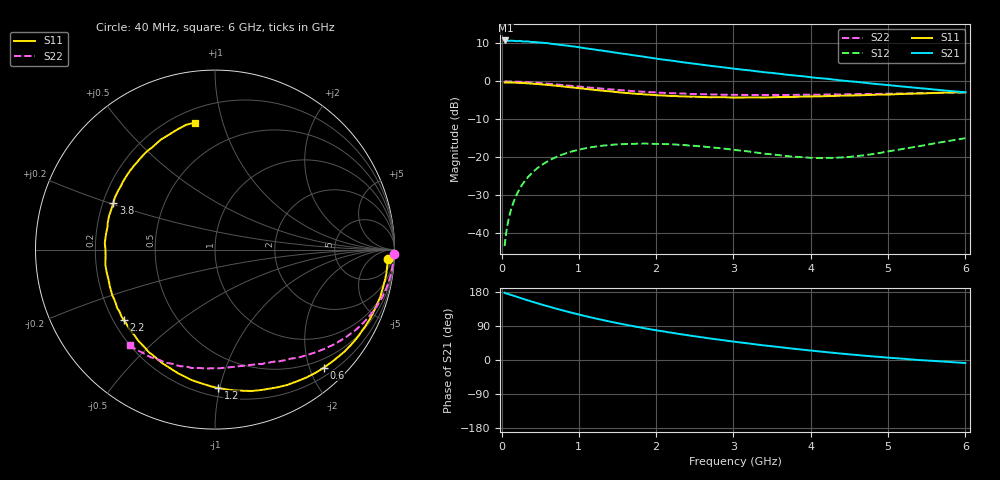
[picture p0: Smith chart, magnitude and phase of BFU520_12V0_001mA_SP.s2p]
! Filename:  P:\Prog\Test\Noise\ATS_data\Testdata_Net\03 Spar\BFU520_APG2013_37_A05_12p0V_001mA_SP_CM01_D.s2p
! Date/Time: Fri 26/Apr/2013 13:00:10
! BFU520_APG2013_37_A05_12p0V_1to20mA_SP_CM01_Bias1_R.s2p
! MDIF S-parameter v. bias file
! BFU520_APG2013_37_A05_12p0V_1to20mA_SP_CM01
! Date/time Tue Apr 23 18:22:57 2013
! bias mode 1
! bias variable = I_out
! VAR bias_var= 1
! VAR V_out= 12.0000
! VAR I_out= 0.9950
! VAR V_in= 0.7863
! VAR I_in= 0.0086
! Device data file deembeded for feedlines and parallel
! Original file: \03 Spar\BFU520_APG2013_37_A05_12p0V_001mA_SP_CM01_R.s2p
! Feed-files: PR047V01_250413_Feed1.s2p, PR047V01_250413_Feed2.s2p
! Parallel-file: PR047V01_250413_Par.s2p
# MHz S MA R 50
!  Freq-MHz  S11-mag  S11-arg  S21-mag  S21-arg  S12-mag  S12-arg  S22-mag  S22-arg
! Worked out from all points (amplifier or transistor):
!   98 points, 40 MHz to 6 GHz, reference 50 ohm
!   highest |S21| = 10.8 dB at 50 MHz (marker M1)
!   |S21| within 3 dB of that: start of sweep to 1.409 GHz
!   unconditionally stable (mu >= 1): 3.535 GHz to 5.175 GHz
!   at 300 MHz: K = 0.08, MSG = 18.4 dB, |S12| = -26.3 dB
!   at 1.6 GHz: K = 0.38, MSG = 11.9 dB, |S12| = -16.5 dB
!   at 6 GHz: K = 0.79, MSG = 6.1 dB, |S12| = -15.0 dB
!   S11 on the Smith chart (normalised r, x): 40 MHz: 16, -26; 600 MHz: 0.34, -2.24; 1.2 GHz: 0.26, -0.99; 2.2 GHz: 0.24, -0.32; 3.8 GHz: 0.24, +0.21; 6 GHz: 0.28, +0.81
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40  0.966 -3.2  3.449 177.6  0.006704 86.5  0.9972 -1.4
50  0.9648 -4.0  3.457 176.3  0.00827 86.2  0.9978 -1.9
80  0.9639 -6.4  3.433 174.6  0.01324 85.2  0.995 -3.3
120  0.9626 -9.7  3.44 171.9  0.01982 83.2  0.9938 -5.1
220  0.9545 -17.7  3.407 165.3  0.03589 78.0  0.9863 -9.4
380  0.9339 -30.4  3.301 154.8  0.05998 69.6  0.9674 -16.2
600  0.8948 -47.3  3.184 141.7  0.08864 59.0  0.9298 -24.6
700  0.8749 -54.8  3.087 135.9  0.09951 54.5  0.9107 -28.2
850  0.8432 -65.4  2.95 127.8  0.1139 48.2  0.8819 -33.0
1050  0.8016 -78.8  2.765 117.5  0.1287 40.6  0.8429 -39.2
1200  0.7716 -88.6  2.63 110.3  0.137 35.5  0.8162 -43.2
1600  0.7028 -112.1  2.291 93.2  0.149 23.7  0.7558 -52.8
1850  0.6721 -125.4  2.101 83.8  0.1512 17.8  0.7286 -57.9
2050  0.6531 -135.3  1.958 76.9  0.149 13.8  0.7075 -61.8
2200  0.6427 -142.5  1.874 72.0  0.1477 11.2  0.698 -64.5
2700  0.6163 -164.8  1.602 56.7  0.1351 4.9  0.6706 -73.6
3100  0.6107 179.6  1.43 46.0  0.1216 3.3  0.6619 -80.4
3800  0.6232 155.2  1.191 29.2  0.1011 10.0  0.6625 -92.6
4100  0.6331 145.7  1.103 22.9  0.09737 16.8  0.6656 -97.8
4700  0.6571 129.1  0.9563 11.3  0.1062 31.7  0.6792 -108.3
5200  0.6831 116.2  0.8506 3.3  0.1289 39.5  0.689 -117.3
6000  0.7166 99.1  0.7172 -8.0  0.1781 41.5  0.7132 -131.9
